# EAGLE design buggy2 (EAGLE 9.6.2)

## Sheet 1 of 2: MCU and power
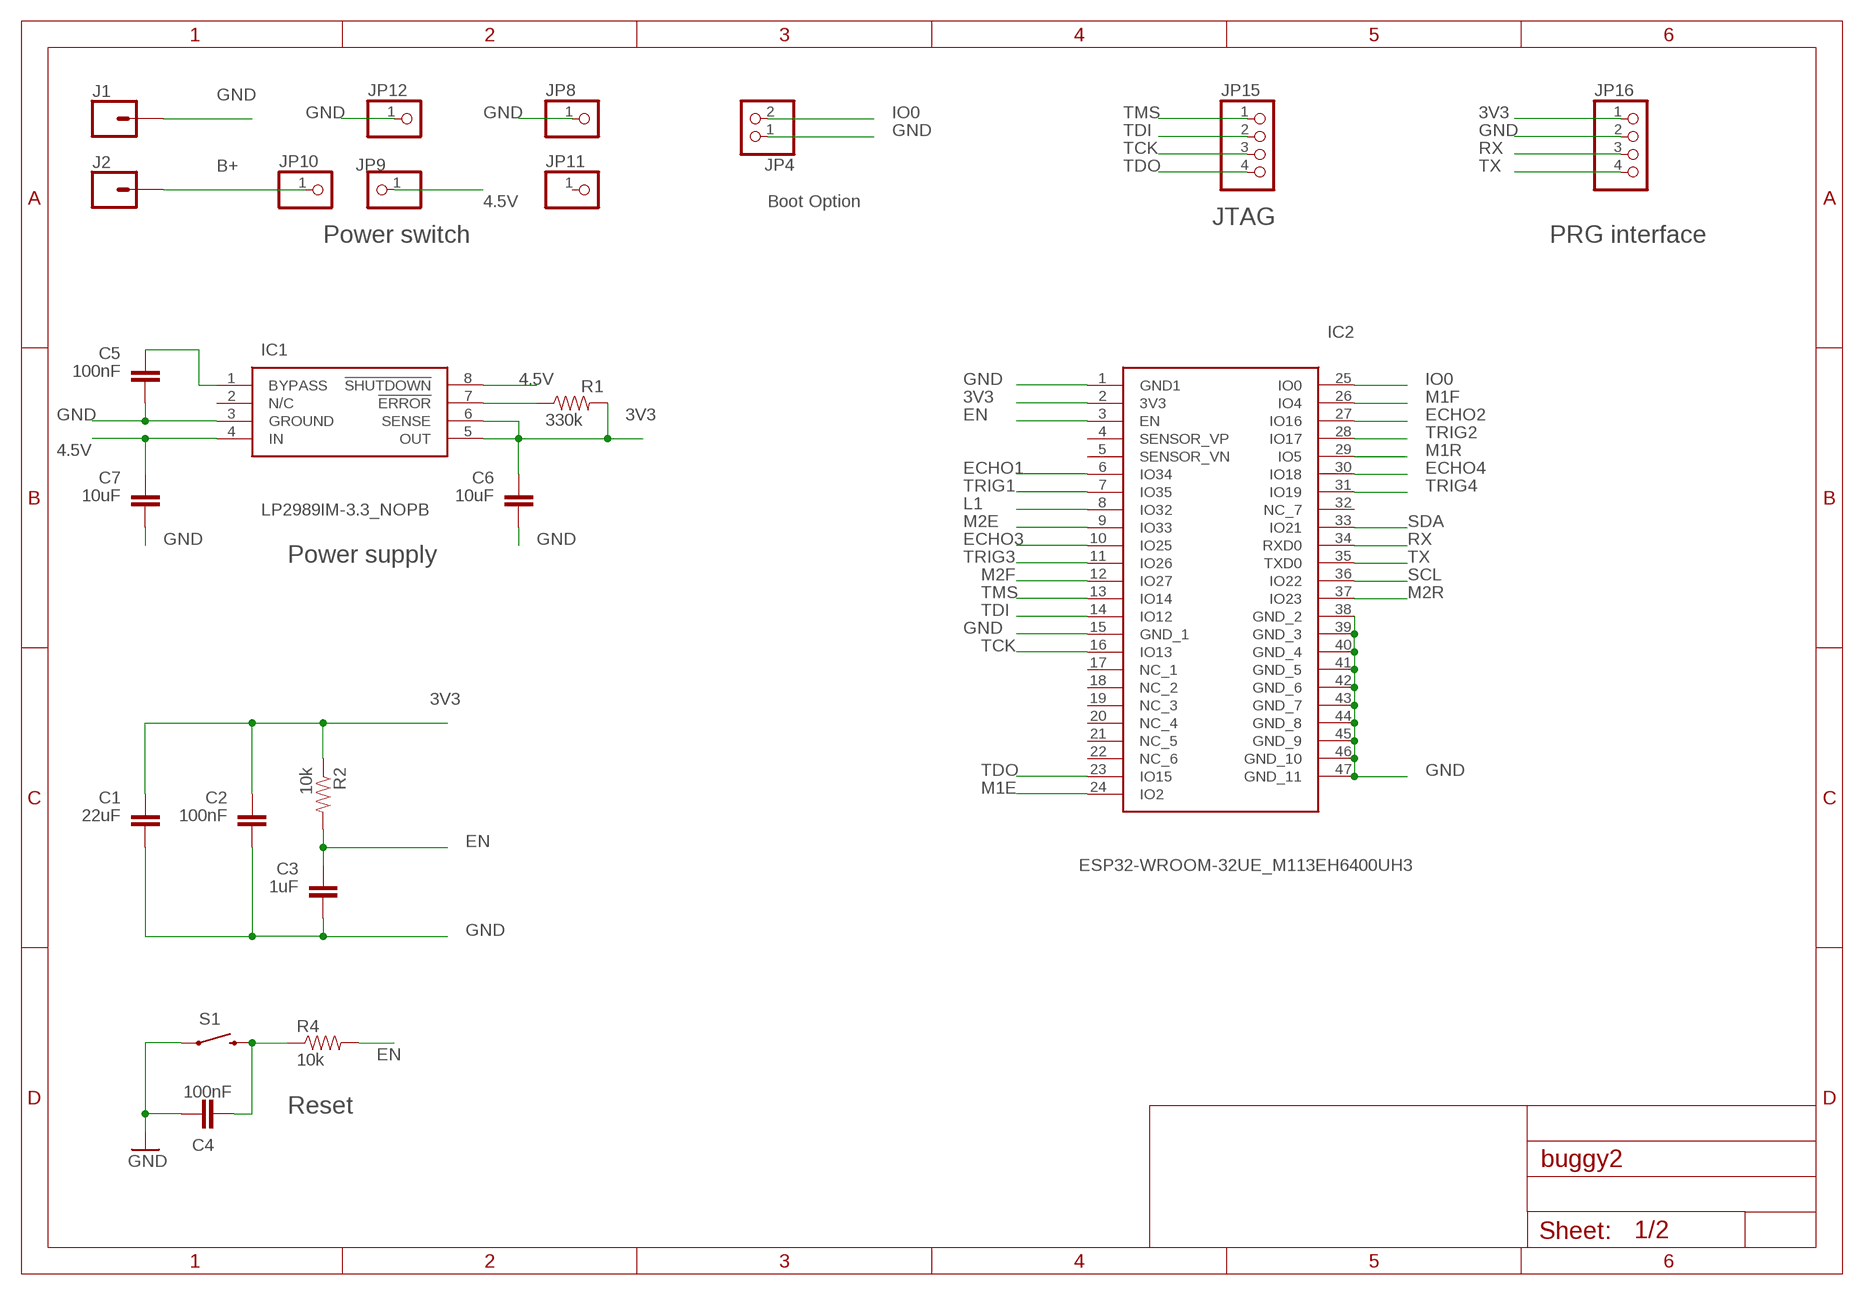
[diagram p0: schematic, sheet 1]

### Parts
C1  22uF  CAP0805  [0805]
C2  100nF  CAP0805  [0805]
C3  1uF  CAP0805  [0805]
C4  100nF  CAP0805  [0805]
C5  100nF  CAP0805  [0805]
C6  10uF  CAP0805  [0805]
C7  10uF  CAP0805  [0805]
IC1  LP2989IM-3.3_NOPB  [SOIC127P600X175-8N]
IC2  ESP32-WROOM-32UE_M113EH6400UH3  [ESP32WROOM32UEM113EH6400UH3Q0]
J1  CONN_01PTH_2MM  [1X01_2MM]
J2  CONN_01PTH_2MM  [1X01_2MM]
JP4  PINHD-1X2  [1X02]
JP8  PINHD-1X1  [1X01]
JP9  PINHD-1X1  [1X01]
JP10  PINHD-1X1  [1X01]
JP11  PINHD-1X1  [1X01]
JP12  PINHD-1X1  [1X01]
JP15  PINHD-1X4  [1X04]
JP16  PINHD-1X4  [1X04]
R1  330k  RESISTOR0805-RES  [0805]
R2  10k  RESISTOR0805-RES  [0805]
R4  10k  RESISTOR0805-RES  [0805]
S1  RESET  SWITCH-MOMENTARY-2SMD-1101NE  [TACTILE-SWITCH-1101NE]

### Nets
3V3: C1.1 C2.1 C6.1 IC1.5(OUT) IC1.6(SENSE) IC2.2(3V3) JP16.1 R1.2 R2.1 ; also sheet 2
4.5V: C7.1 IC1.4(IN) IC1.8(!SHUTDOWN) JP9.1 ; also sheet 2
B+: J2.1 JP10.1
ECHO1: IC2.6(IO34) ; also sheet 2
ECHO2: IC2.27(IO16) ; also sheet 2
ECHO3: IC2.10(IO25) ; also sheet 2
ECHO4: IC2.30(IO18) ; also sheet 2
EN: C3.1 IC2.3(EN) R2.2 R4.2
GND: C1.2 C2.2 C3.2 C4.1 C5.2 C6.2 C7.2 IC1.3(GROUND) IC2.1(GND1) IC2.15(GND_1) IC2.38(GND_2) IC2.39(GND_3) IC2.40(GND_4) IC2.41(GND_5) IC2.42(GND_6) IC2.43(GND_7) IC2.44(GND_8) IC2.45(GND_9) IC2.46(GND_10) IC2.47(GND_11) J1.1 JP4.1 JP8.1 JP12.1 JP16.2 S1.1 ; also sheet 2
IO0: IC2.25(IO0) JP4.2
L1: IC2.8(IO32) ; also sheet 2
M1E: IC2.24(IO2) ; also sheet 2
M1F: IC2.26(IO4) ; also sheet 2
M1R: IC2.29(IO5) ; also sheet 2
M2E: IC2.9(IO33) ; also sheet 2
M2F: IC2.12(IO27) ; also sheet 2
M2R: IC2.37(IO23) ; also sheet 2
N$1: C5.1 IC1.1(BYPASS)
N$3: C4.2 R4.1 S1.2
N$18: IC1.7(!ERROR) R1.1
RX: IC2.34(RXD0) JP16.3
SCL: IC2.36(IO22) ; also sheet 2
SDA: IC2.33(IO21) ; also sheet 2
TCK: IC2.16(IO13) JP15.3
TDI: IC2.14(IO12) JP15.2
TDO: IC2.23(IO15) JP15.4
TMS: IC2.13(IO14) JP15.1
TRIG1: IC2.7(IO35) ; also sheet 2
TRIG2: IC2.28(IO17) ; also sheet 2
TRIG3: IC2.11(IO26) ; also sheet 2
TRIG4: IC2.31(IO19) ; also sheet 2
TX: IC2.35(TXD0) JP16.4
Unconnected: IC1.2(N/C) IC2.4(SENSOR_VP) IC2.5(SENSOR_VN) IC2.17(NC_1) IC2.18(NC_2) IC2.19(NC_3) IC2.20(NC_4) IC2.21(NC_5) IC2.22(NC_6) IC2.32(NC_7) JP11.1

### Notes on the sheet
- Boot Option
- JTAG
- Power switch | PRG interface
- Power supply
- Reset

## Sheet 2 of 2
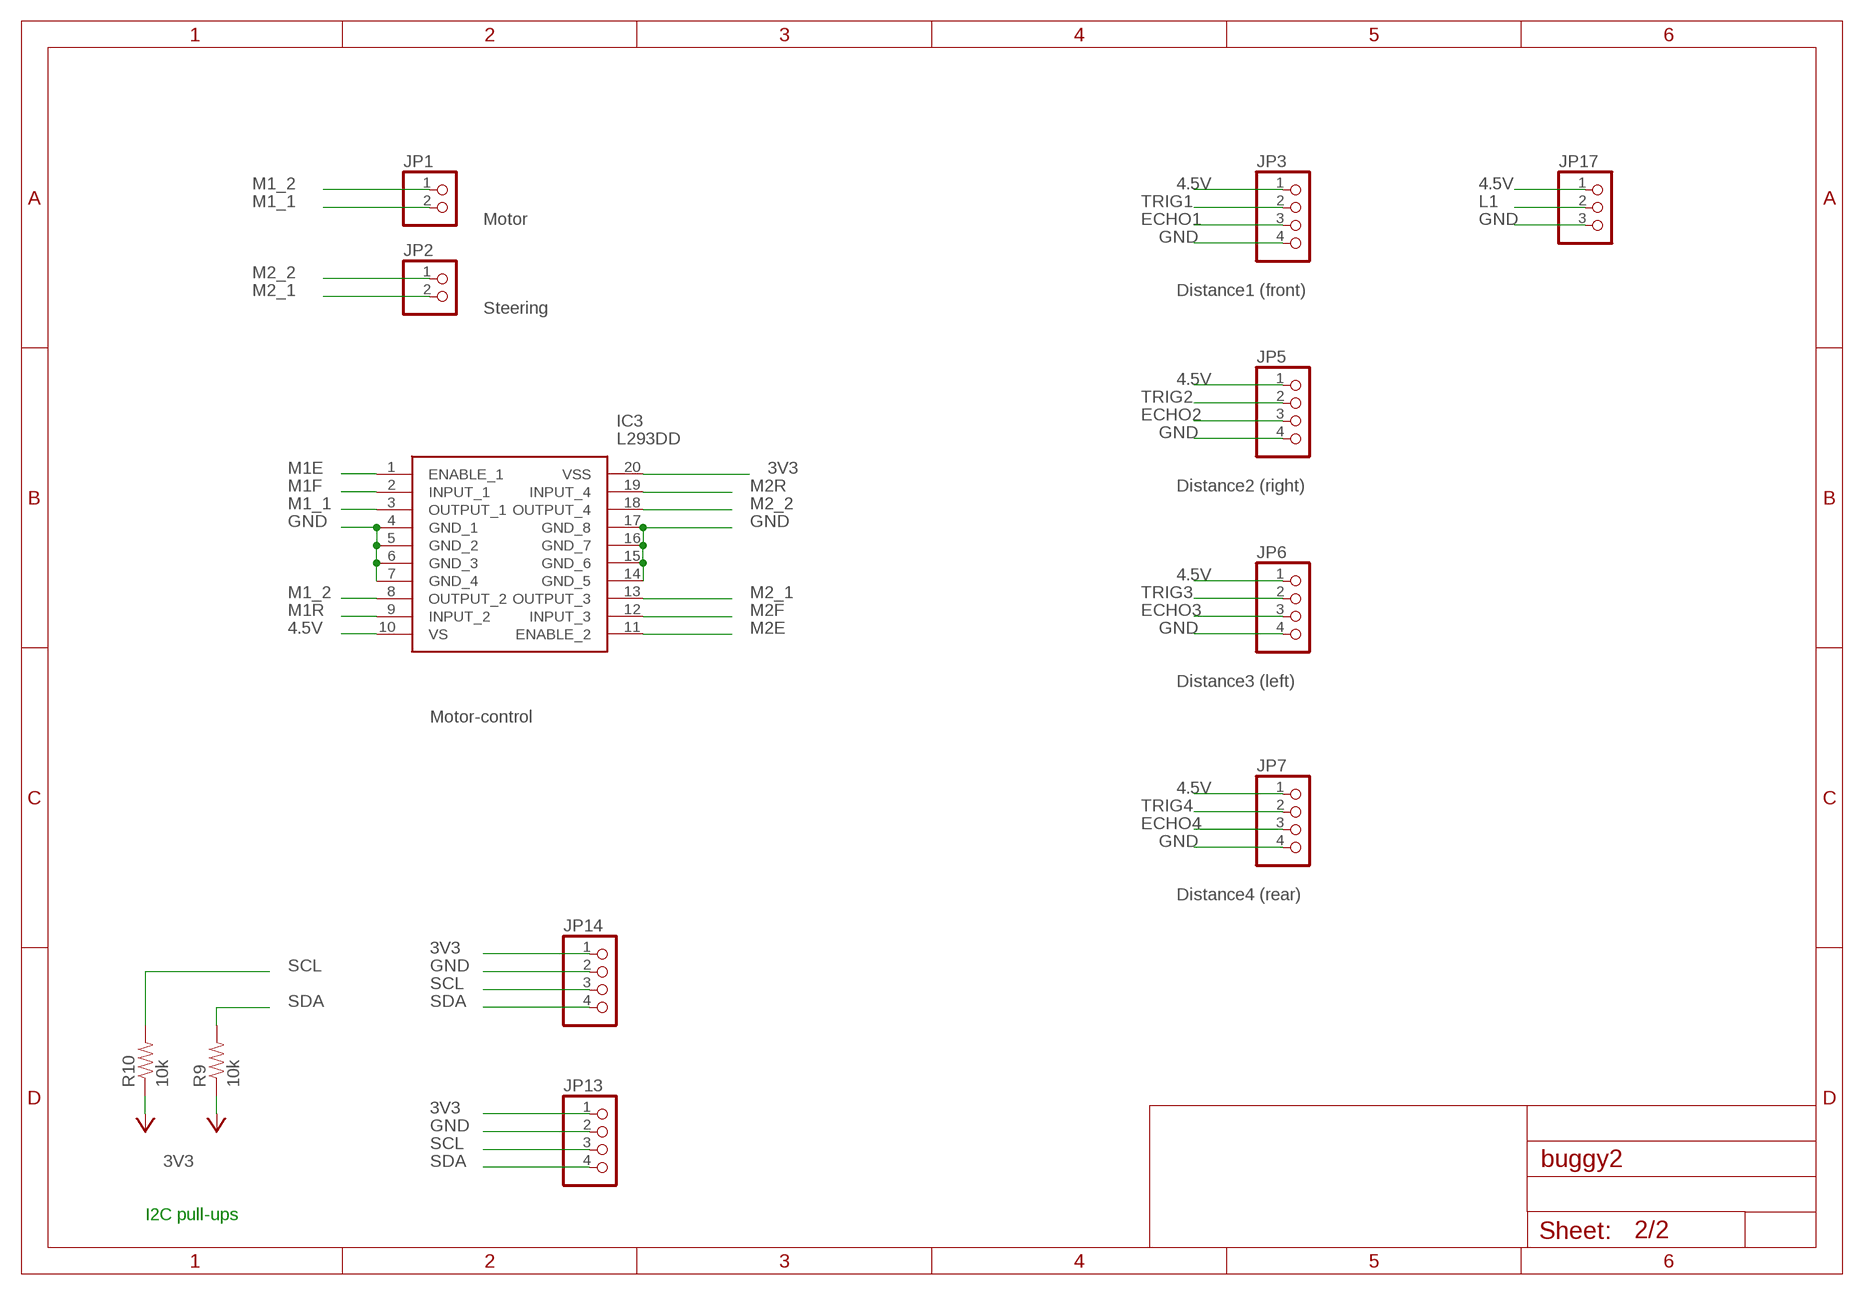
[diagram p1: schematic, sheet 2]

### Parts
IC3  L293DD  [SOIC127P1032X265-20N]
JP1  PINHD-1X2/90  [1X02/90]
JP2  PINHD-1X2/90  [1X02/90]
JP3  PINHD-1X4  [1X04]
JP5  PINHD-1X4  [1X04]
JP6  PINHD-1X4  [1X04]
JP7  PINHD-1X4  [1X04]
JP13  PINHD-1X4  [1X04]
JP14  PINHD-1X4  [1X04]
JP17  PINHD-1X3  [1X03]
R9  10k  RESISTOR0805-RES  [0805]
R10  10k  RESISTOR0805-RES  [0805]

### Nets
3V3: IC3.20(VSS) JP13.1 JP14.1 R9.1 R10.1 ; supply symbol labelled +3V3 ; also sheet 1
4.5V: IC3.10(VS) JP3.1 JP5.1 JP6.1 JP7.1 JP17.1 ; also sheet 1
ECHO1: JP3.3 ; also sheet 1
ECHO2: JP5.3 ; also sheet 1
ECHO3: JP6.3 ; also sheet 1
ECHO4: JP7.3 ; also sheet 1
GND: IC3.4(GND_1) IC3.5(GND_2) IC3.6(GND_3) IC3.7(GND_4) IC3.14(GND_5) IC3.15(GND_6) IC3.16(GND_7) IC3.17(GND_8) JP3.4 JP5.4 JP6.4 JP7.4 JP13.2 JP14.2 JP17.3 ; also sheet 1
L1: JP17.2 ; also sheet 1
M1_1: IC3.3(OUTPUT_1) JP1.2
M1_2: IC3.8(OUTPUT_2) JP1.1
M1E: IC3.1(ENABLE_1) ; also sheet 1
M1F: IC3.2(INPUT_1) ; also sheet 1
M1R: IC3.9(INPUT_2) ; also sheet 1
M2_1: IC3.13(OUTPUT_3) JP2.2
M2_2: IC3.18(OUTPUT_4) JP2.1
M2E: IC3.11(ENABLE_2) ; also sheet 1
M2F: IC3.12(INPUT_3) ; also sheet 1
M2R: IC3.19(INPUT_4) ; also sheet 1
SCL: JP13.3 JP14.3 R10.2 ; also sheet 1
SDA: JP13.4 JP14.4 R9.2 ; also sheet 1
TRIG1: JP3.2 ; also sheet 1
TRIG2: JP5.2 ; also sheet 1
TRIG3: JP6.2 ; also sheet 1
TRIG4: JP7.2 ; also sheet 1

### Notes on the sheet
- Motor
- Distance1 (front)
- Steering
- Distance2 (right)
- Distance3 (left)
- Motor-control
- Distance4 (rear)
- I2C pull-ups

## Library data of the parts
C1-C7 = SparkFun-Passives:CAP: Capacitor
IC1 = SamacSys_Parts:LP2989IM-3.3_NOPB: Micropower/Low Noise, 500 mA Ultra Low-Dropout Regulator Source: Datasheet; DESCRIPTION: Micropower/Low Noise, 500 mA Ultra Low-Dropout Regulator; HEIGHT: 1.75mm; MANUFACTURER_NAME: Texas Instruments; MANUFACTURER_PART_NUMBER: LP2989IM-3.3/NOPB; MOUSER_PART_NUMBER: 926-2989IM-3.3/NOPB; MOUSER_PRICE-STOCK: https://www.mouser.co.uk/ProductDetail/Texas-Instruments/LP2989IM-33-NOPB?qs=1FNqv8aZn1Tm79MYQqSiDQ%3D%3D
IC2 = SamacSys_Parts:ESP32-WROOM-32UE_M113EH6400UH3: WiFi Modules (802.11) SMD module ESP32-WROOM-32UE, ESP32-D0WD-V3, ESP32 ECO V3, 8 MB SPI flash, IPEX antenna connector Source: Datasheet; DESCRIPTION: WiFi Modules (802.11) SMD module ESP32-WROOM-32UE, ESP32-D0WD-V3, ESP32 ECO V3, 8 MB SPI flash, IPEX antenna connector; HEIGHT: 3.35mm; MANUFACTURER_NAME: Espressif Systems; MANUFACTURER_PART_NUMBER: ESP32-WROOM-32UE(M113EH6400UH3Q0); MOUSER_PART_NUMBER: 356-ESP32WRM32UE64UH; MOUSER_PRICE-STOCK: https://www.mouser.co.uk/ProductDetail/Espressif-Systems/ESP32-WROOM-32UEM113EH6400UH3Q0?qs=vHuUswq2%252BsxjtHWnhz9C5Q%3D%3D
IC3 = SamacSys_Parts:L293DD: L293DD, Motor Driver, 4.5 36 V, 20-Pin SOIC Source: Datasheet; DESCRIPTION: L293DD, Motor Driver, 4.5 36 V, 20-Pin SOIC; HEIGHT: 2.65mm; MANUFACTURER_NAME: STMicroelectronics; MANUFACTURER_PART_NUMBER: L293DD; MOUSER_PART_NUMBER: 511-L293DD; MOUSER_PRICE-STOCK: https://www.mouser.co.uk/ProductDetail/STMicroelectronics/L293DD?qs=m4gxtLzGBzoksItTiSkcgg%3D%3D
J1 J2 = SparkFun-Connectors:CONN_01: Single connection point. Often used as Generic Header-pin footprint for 0.1 inch spaced/style header connections
JP1 JP2 JP4 = pinhead:PINHD-1X2: PIN HEADER
JP3 JP5-JP7 JP13-JP16 = pinhead:PINHD-1X4: PIN HEADER
JP8-JP12 = pinhead:PINHD-1X1: PIN HEADER
JP17 = pinhead:PINHD-1X3: PIN HEADER
R1 R2 R4 R9 R10 = SparkFun-Resistors:RESISTOR: Resistor
S1 = SparkFun-Electromechanical:SWITCH-MOMENTARY-2: Various NO switches- pushbuttons, reed, etc; PROD_ID: SWCH-00815

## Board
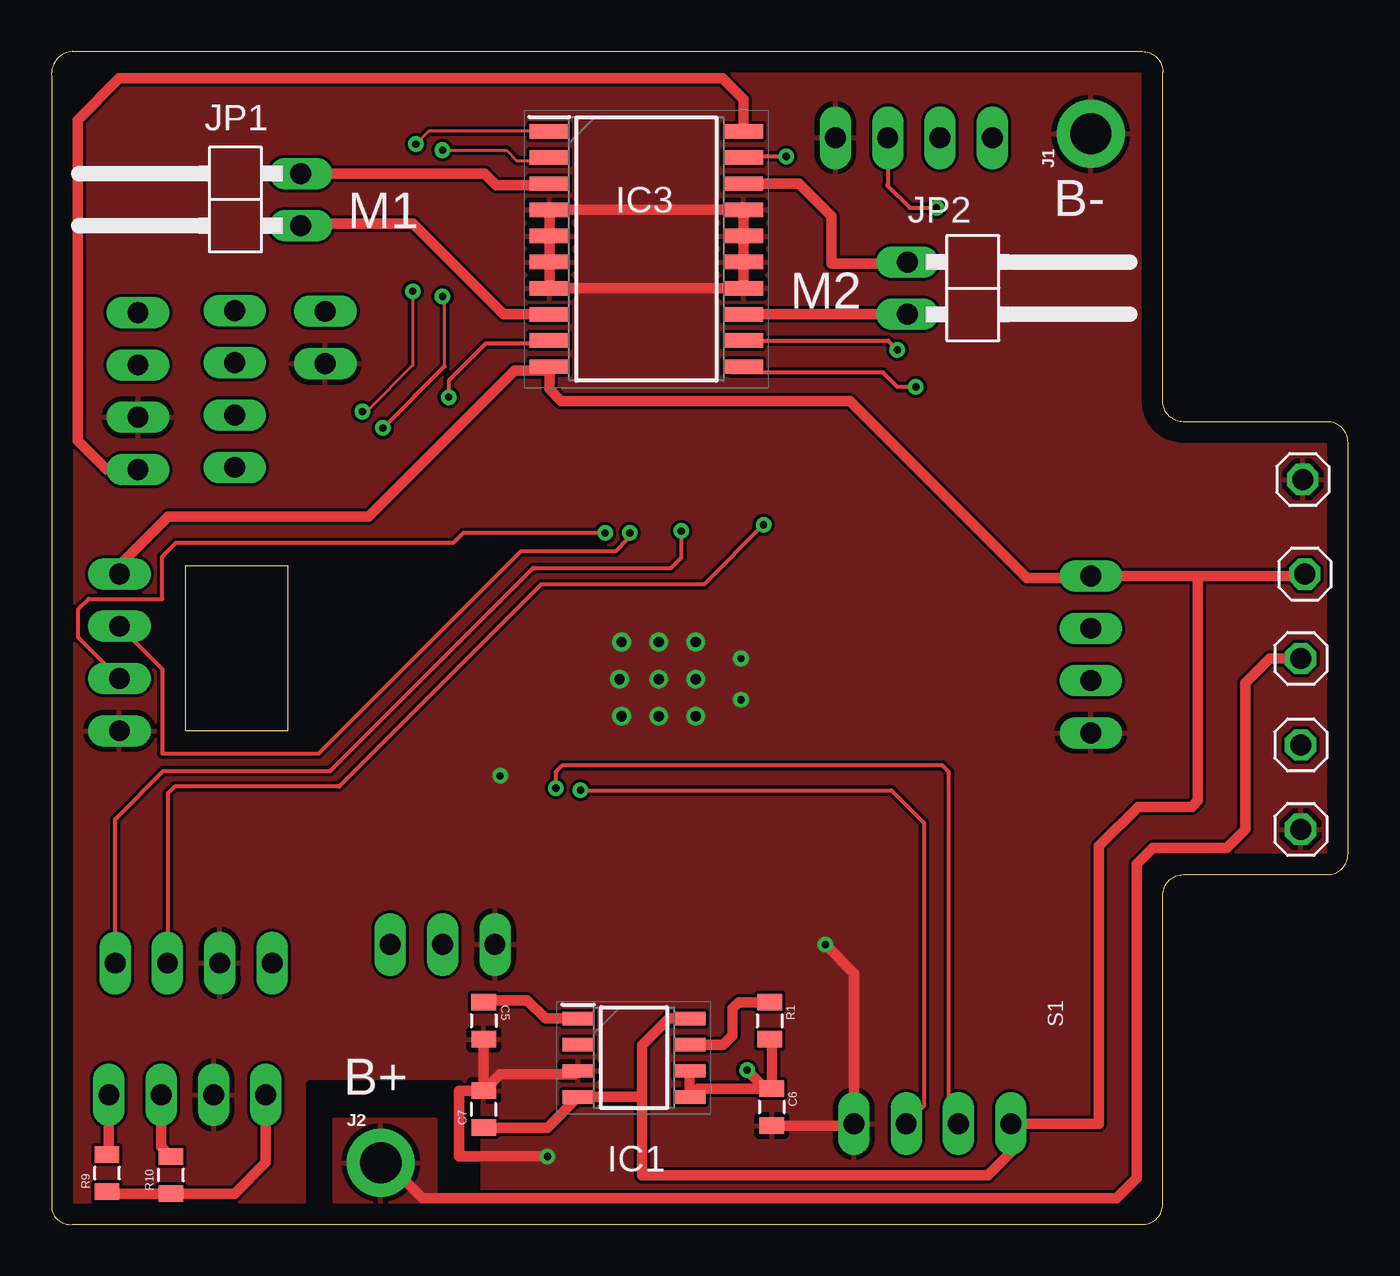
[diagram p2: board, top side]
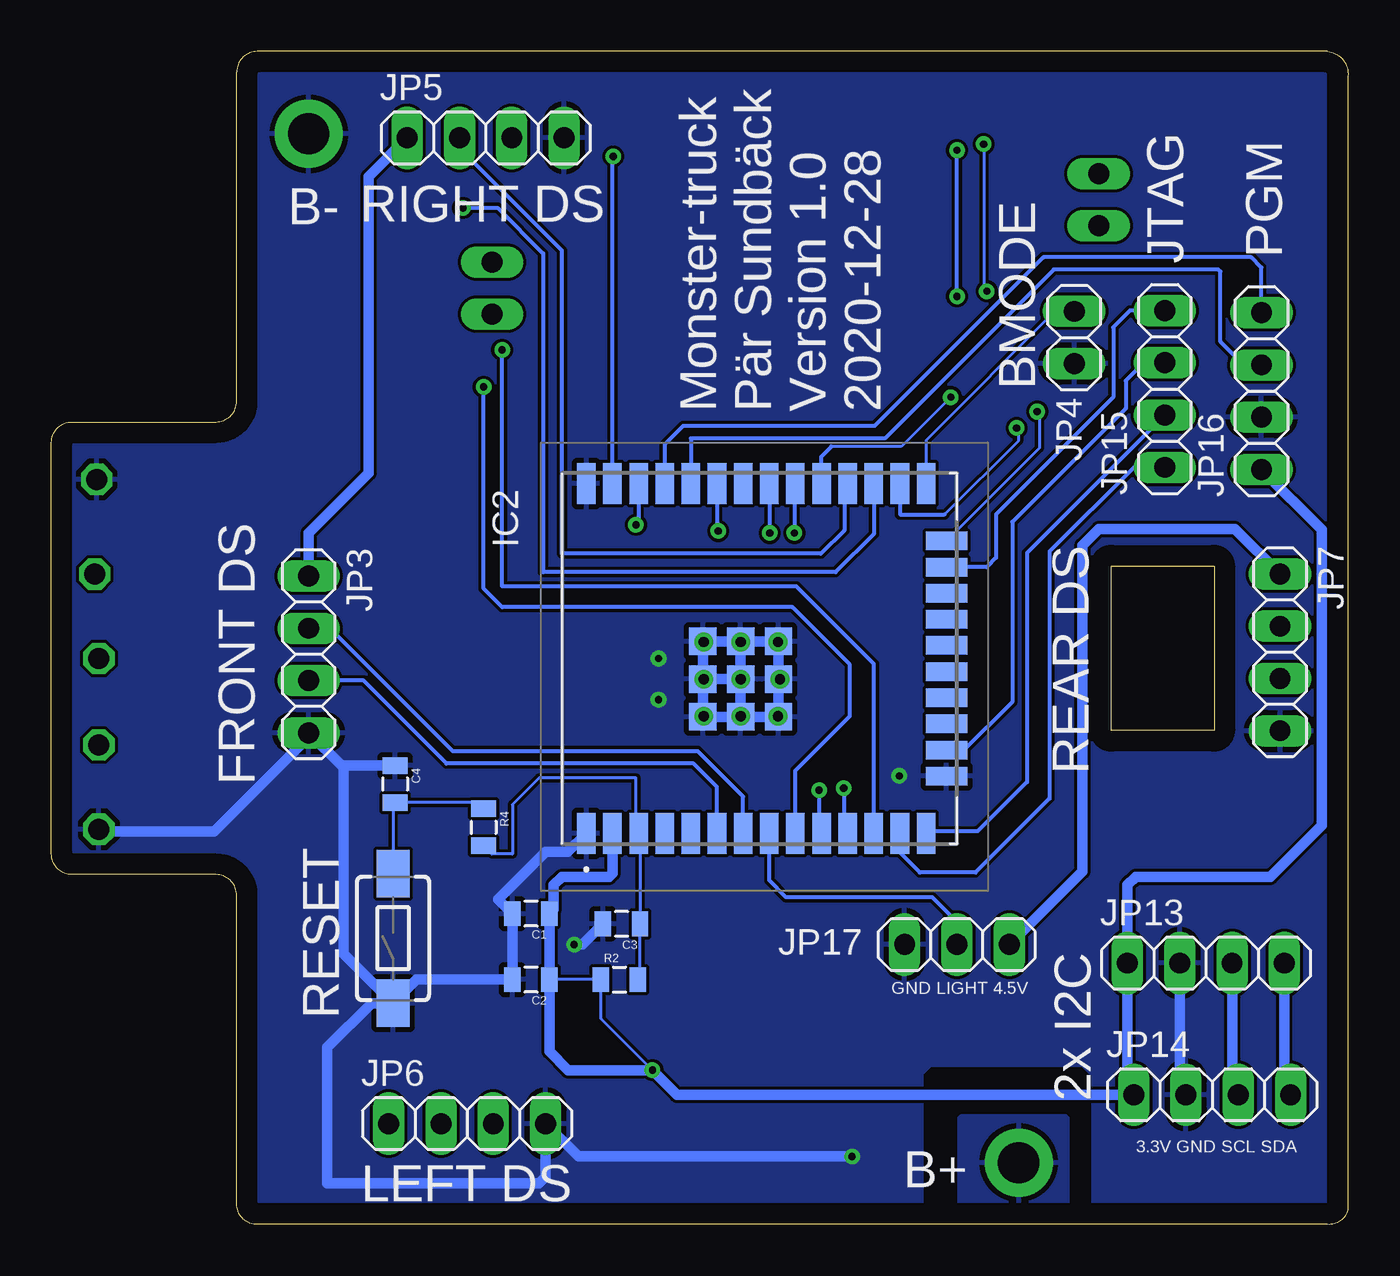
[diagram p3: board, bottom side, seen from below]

Size 63 x 57.01 mm. Coordinates in mm from the lower left corner, seen from the top.
Outline: 0,55.81 0,0.81 arc90 1,0.01 53,0.01 arc90 54,1.01 54,16.01 arc-90 55,17.01 62,17.01 arc90 63,18.01 63,38.01 arc90 62,39.01 55,39.01 arc-90 54,40.01 54,56.01 arc90 53,57.01 1,57.01 arc90 0,55.81
Outline: 6.5,32.01 6.5,24.01 11.5,24.01 11.5,32.01 6.5,32.01
Copper layers (1*16): Top 0.035mm / dielectric 1.5mm / Bottom 0.035mm
Design rules "default": minimum track width 6mil, minimum drill 0.35mm, track to track 6mil, track to pad 6mil, pad to pad 6mil, via to via 6mil, smd to smd 6mil, copper to edge 40mil, drill to drill 6mil, minimum pad ring 10mil, minimum via ring 8mil, stop-mask expansion 4mil, vias tented up to drill 0mil, thermal gap 10mil

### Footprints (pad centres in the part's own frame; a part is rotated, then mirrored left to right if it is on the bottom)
0805 = smd 0.8 x 1.2: 1 -0.9,0; 2 0.9,0
SOIC127P600X175-8N = smd 1.528 x 0.65: 1 -2.711,1.905; 2 -2.711,0.635; 3 -2.711,-0.635; 4 -2.711,-1.905; 5 2.711,-1.905; 6 2.711,-0.635; 7 2.711,0.635; 8 2.711,1.905
ESP32WROOM32UEM113EH6400UH3Q0 = smd 2 x 0.9: 1 -8.5,8.41; 2 -8.5,7.14; 3 -8.5,5.87; 4 -8.5,4.6; 5 -8.5,3.33; 6 -8.5,2.06; 7 -8.5,0.79; 8 -8.5,-0.48; 9 -8.5,-1.75; 10 -8.5,-3.02; 11 -8.5,-4.29; 12 -8.5,-5.56; 13 -8.5,-6.83; 14 -8.5,-8.1; 25 8.5,-8.1; 26 8.5,-6.83; 27 8.5,-5.56; 28 8.5,-4.29; 29 8.5,-3.02; 30 8.5,-1.75; 31 8.5,-0.48; 32 8.5,0.79; 33 8.5,2.06; 34 8.5,3.33; 35 8.5,4.6; 36 8.5,5.87; 37 8.5,7.14; 38 8.5,8.41 | smd 0.9 x 2: 15 -5.715,-9.1; 16 -4.445,-9.1; 17 -3.175,-9.1; 18 -1.905,-9.1; 19 -0.635,-9.1; 20 0.635,-9.1; 21 1.905,-9.1; 22 3.175,-9.1; 23 4.445,-9.1; 24 5.715,-9.1 | smd 1.33 x 1.33: 39 -1,0.91; 40 0.835,0.91; 41 0.835,2.745; 42 -1,2.745; 43 -2.835,2.745; 44 -2.835,0.91; 45 -2.835,-0.925; 46 -1,-0.925; 47 0.835,-0.925
SOIC127P1032X265-20N = smd 1.925 x 0.7: 1 -4.712,5.715; 2 -4.712,4.445; 3 -4.712,3.175; 4 -4.712,1.905; 5 -4.712,0.635; 6 -4.712,-0.635; 7 -4.712,-1.905; 8 -4.712,-3.175; 9 -4.712,-4.445; 10 -4.712,-5.715; 11 4.712,-5.715; 12 4.712,-4.445; 13 4.712,-3.175; 14 4.712,-1.905; 15 4.712,-0.635; 16 4.712,0.635; 17 4.712,1.905; 18 4.712,3.175; 19 4.712,4.445; 20 4.712,5.715
1X01_2MM = drill 2 pad 3.302: 1 0,0
1X02/90 = drill 1.016 long: 1 -1.27,-3.81; 2 1.27,-3.81
1X04 = drill 1.016 long: 1 -3.81,0; 2 -1.27,0; 3 1.27,0; 4 3.81,0
1X02 = drill 1.016 long: 1 -1.27,0; 2 1.27,0
1X01 = drill 1.016 octagon: 1 0,0
1X03 = drill 1.016 long: 1 -2.54,0; 2 0,0; 3 2.54,0
TACTILE-SWITCH-1101NE = smd 2.3 x 1.6: 1 -3.15,0; 2 3.15,0

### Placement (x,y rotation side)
C1  39.7,15.11 180 bottom
C2  39.7,11.91 180 bottom
C3  35.3,14.61 180 bottom
C4  46.3,21.41 270 bottom
C5  21,9.91 270.3 top
C6  35,5.71 270 top
C7  21,5.61 90 top
IC1  28.3,8.11 0 top
IC2  28.6,27.51 90 bottom
IC3  28.9,47.41 0 top
J1  50.5,53.01 90 top
J2  16,3.01 0 top
JP1  8.3,49.81 90 top
JP2  45.4,45.51 270 top
JP3  50.5,27.71 270 bottom
JP4  13.3,43.11 90 bottom
JP5  41.9,52.81 0 bottom
JP6  42.8,4.91 0 bottom
JP7  3.3,27.81 270 bottom
JP8  60.8,36.21 0 top
JP9  60.9,31.61 0 top
JP10  60.7,27.51 0 top
JP11  60.7,23.31 0 top
JP12  60.7,19.21 0 top
JP13  6.9,12.71 0 bottom
JP14  6.6,6.31 0 bottom
JP15  8.9,40.61 90 bottom
JP16  4.2,40.51 90 bottom
JP17  19,13.61 180 bottom
R1  34.9,9.91 270 top
R2  35.4,11.91 0 bottom
R4  42,19.31 270 bottom
R9  2.7,2.51 90 top
R10  5.8,2.41 90 top
S1  46.4,13.91 90 bottom

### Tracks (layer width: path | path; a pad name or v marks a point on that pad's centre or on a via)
3V3  (via drill 0.35)
  Top 0.508: IC1.6 IC1.5 31.42,6.61 C6.1 | R1.2 35,8.91 C6.1 | v33.8,7.51 34.7,6.61 C6.1 | R9.1 2.8,1.51 R10.1 8.9,1.51 10.41,3.02 JP14.1 | JP16.1 2.68,36.7 1.27,38.11 1.27,53.68 3.3,55.71 32.6,55.71 33.62,54.69 IC3.20
  Bottom 0.152: 38.8,12.01 C2.1 R2.1 36.3,10.01 v33.8,7.51
  Bottom 0.508: 38.8,12.01 38.8,8.41 37.9,7.51 v33.8,7.51 32.6,6.31 JP14.1 10.71,6.61 JP13.1 10.71,16.5 10.3,16.91 3.77,16.91 1.27,19.41 1.27,33.77 JP16.1 | C2.1 C1.1 38.6,15.31 38.6,16.51 38.2,16.91 35.9,16.91 35.74,17.07 IC2.2
4.5V
  Top 0.508: 28.7,6.21 28.7,2.41 45.51,2.41 46.61,3.51 JP6.1 50.9,4.91 50.9,18.41 52.8,20.31 55.4,20.31 55.7,20.61 55.7,31.52 | 28.7,6.21 28.7,8.71 30.01,10.01 IC1.8 | 28.7,6.21 IC1.4 24.1,4.71 C7.1 | IC3.10 24.19,41.51 | 24.19,41.51 24.19,40.59 24.77,40.01 38.8,40.01 47.4,31.41 50.39,31.41 JP3.1 55.7,31.52 | JP7.1 3.23,31.69 3.23,31.98 5.66,34.41 15.4,34.41 22.5,41.51 24.19,41.51 | 55.7,31.52 60.81,31.52 JP9.1
  Bottom 0.508: JP5.1 47.6,50.92 47.6,36.51 50.5,33.61 JP3.1 | JP17.1 12.9,17.17 12.9,33.01 12.1,33.81 5.49,33.81 JP7.1
B+
  Top 0.508: J2.1 16.3,3.01 18.03,1.28 51.73,1.28 52.73,2.28 52.73,17.53 53.51,18.31 57.1,18.31 58,19.21 58,26.31 59.2,27.51 JP10.1
  pour Top: 13.7,5.11 13.7,1.11 18.7,1.11 18.7,5.11
  pour Bottom: 13.6,5.21 13.6,0.91 18.8,0.91 18.9,1.01 18.9,5.21 18.8,5.31 13.7,5.31
ECHO1
  Bottom 0.2: IC2.6 30.66,21.27 31.8,22.41 43.8,22.41 47.83,26.44 JP3.3
ECHO2  (via drill 0.35)
  Top 0.2: JP5.3 40.63,50.54 40.6,50.51 41.7,49.41 v43,49.41
  Bottom 0.2: IC2.27 23.04,33.57 24.9,31.71 39.1,31.71 39.1,47.18 41.33,49.41 v43,49.41
ECHO3  (via drill 0.35)
  Top 0.2: v25.7,21.11 40.8,21.11 42.4,19.51 42.4,5.78 JP6.3
  Bottom 0.2: v25.7,21.11 25.7,19.13 IC2.10
ECHO4  (via drill 0.35)
  Top 0.2: JP7.3 1.3,28.54 1.3,29.91 1.8,30.41 5.39,30.41 5.39,32.47 6.04,33.12 19.52,33.12 20,33.61 v26.9,33.61
  Bottom 0.2: IC2.30 26.9,35.96 v26.9,33.61
EN
  Bottom 0.152: R2.2 34.4,12.01 C3.1 34.4,19.01 IC2.3 34.6,19.14 34.6,21.71 39.3,21.71 40.6,20.41 40.6,18.01 41.6,18.01 R4.2
GND  (via drill 0.35, 0.5)
  Top 0.508: C5.2 C7.2 | C7.2 19.8,6.51 19.8,3.31 v24.1,3.31 | IC1.3 25.43,7.31 21.8,7.31 C7.2 | C6.2 38.89,4.81 JP6.4 38.99,12.22 v37.6,13.61 | IC3.4 IC3.5 IC3.6 IC3.7 IC3.14 IC3.15 IC3.16 IC3.17 IC3.4
  Bottom 0.508: JP13.2 8.17,6.61 JP14.2 | S1.1 47.45,10.76 49.6,8.61 49.6,2.01 39.3,2.01 38.99,2.32 JP6.4 37.39,3.31 v24.1,3.31 | S1.1 45.25,11.91 C2.2 C1.2 41.3,15.81 39,18.11 37.91,18.11 IC2.1 | 48.8,22.31 48.91,22.31 JP3.4 50.5,23.71 55.1,19.11 60.6,19.11 JP12.1 | 48.8,22.31 C4.1 | v37.6,13.61 37.2,13.61 C3.2 | S1.1 48.8,13.16 48.8,22.31 | IC2.40 IC2.47 IC2.46 IC2.45 IC2.44 | IC2.40 IC2.41 IC2.42 | IC2.42 IC2.43 IC2.44 | IC2.39 IC2.44 | IC2.40 IC2.39 | IC2.39 IC2.42
  other vias: 21.8,21.81 31.3,28.31 27.6,26.51 27.7,28.31 29.5,28.31 29.5,26.51 31.3,26.51 27.7,24.71 29.5,24.71 31.3,24.71 33.5,27.51 33.5,25.51
  pour Top: -1.1,56.31 -1.1,0.81 0.7,-0.99 10.6,-0.99 10.9,-0.69 12.3,0.71 12.3,6.91 12.5,7.11 19.9,7.11 20.9,6.11 20.9,-0.59 21.4,-1.09 54.3,-1.09 64.6,9.21 64.6,54.11 60.7,58.01 0.1,58.01 -1.1,56.81
  pour Bottom: -2,57.31 -2,-1.19 -2.1,-1.29 12.1,-1.29 12.4,-0.99 12.4,7.21 12.9,7.71 20.3,7.71 20.7,7.31 20.7,-1.29 56.1,-1.29 56.4,-0.99 64.6,7.21 64.6,24.11 64.6,57.01 62.9,58.71 -0.6,58.71
IO0
  Bottom 0.152: JP4.2 14.23,44.38 20.5,38.11 IC2.25
L1
  Bottom 0.2: JP17.2 19,14.71 20.2,15.91 27.3,15.91 28.12,16.73 IC2.8
M1_1
  Top 0.508: JP1.2 21.03,51.08 21.6,50.51 24.12,50.51 IC3.3
M1_2
  Top 0.508: IC3.8 21.98,44.23 17.57,48.64 12.21,48.64 JP1.1
M1E  (via drill 0.35)
  Top 0.152: IC3.1 18.32,53.12 v17.7,52.51 | v17.55,45.36 17.55,41.76 15.3,39.51 v15.1,39.51
  Bottom 0.152: v17.7,52.51 17.7,45.41 17.6,45.31 v17.55,45.36 | v15.1,39.51 15,39.41 15,37.72 IC2.24
M1F  (via drill 0.35)
  Top 0.152: 19.1,41.71 19.1,45.11 v19,45.11 | v19,52.21 22.1,52.21 22.6,51.71 24.05,51.71 IC3.2
  Top 0.2: v16.1,38.71 19.1,41.71
  Bottom 0.152: v16.1,38.71 16,38.61 16,38.11 19.6,34.51
  Bottom 0.2: IC2.26 21.77,34.51 19.6,34.51 | v19,45.11 v19,52.21
M1R  (via drill 0.35)
  Top 0.152: IC3.9 24.04,42.81
  Top 0.2: 24.04,42.81 21.1,42.81 19.3,41.01 v19.3,40.21
  Bottom 0.152: v19.3,40.21 21.7,37.81 25.1,37.81 | 25.6,36.03 IC2.29
  Bottom 0.2: 25.1,37.81 25.6,37.31 25.6,36.03
M2_1
  Top 0.508: IC3.13 37.59,44.23 37.59,44.24 JP2.2
M2_2
  Top 0.508: IC3.18 36.33,50.58 37.9,49.01 37.9,46.71 41.52,46.71 JP2.1
M2E  (via drill 0.35)
  Top 0.2: v42,40.71 41.1,40.71 40.4,41.41 33.03,41.41 33.32,41.69 IC3.11
  Bottom 0.2: IC2.9 26.85,22.06 24.2,24.71 24.2,27.21 27,30.01 41.1,30.01 42,30.91 v42,40.71
M2F  (via drill 0.35)
  Top 0.2: IC3.12 40.65,42.96 v41.1,42.51
  Bottom 0.2: IC2.12 23.04,27.25 26.8,31.01 41.1,31.01 v41.1,42.51
M2R  (via drill 0.35)
  Top 0.2: IC3.19 33.67,51.91 v35.7,51.91
  Bottom 0.2: IC2.37 35.74,51.87 v35.7,51.91
N$1
  Top 0.508: IC1.1 24,10.01 23.1,10.91 21.1,10.91 C5.1
N$3
  Bottom 0.152: S1.2 46.4,20.41 C4.2 42.3,20.51 R4.1
N$18
  Top 0.508: IC1.7 32.64,8.74 33.1,9.21 33.1,10.51 33.4,10.81 R1.1
RX
  Bottom 0.2: JP16.3 5.07,41.78 6.2,42.91 6.2,46.31 6.3,46.41 14.3,46.41 22.5,38.21 31.93,38.21 IC2.34
SCL  (via drill 0.35)
  Top 0.2: v34.6,34.01 31.7,31.11 23.8,31.11 13.98,21.28 5.98,21.28 5.65,20.96 5.65,12.73 JP13.3
  Top 0.508: JP14.3 5.33,3.78 R10.2
  Bottom 0.2: IC2.36 34.47,34.14 v34.6,34.01
  Bottom 0.508: JP13.3 5.63,6.61 JP14.3
SDA  (via drill 0.35)
  Top 0.2: JP13.4 3.09,19.7 5.44,22.04 13.53,22.04 23.4,31.91 30.1,31.91 30.6,32.41 v30.6,33.71
  Top 0.508: JP14.4 2.79,3.5 R9.2
  Bottom 0.2: IC2.33 30.66,33.77 v30.6,33.71
  Bottom 0.508: JP13.4 3.09,6.61 JP14.4
TCK
  Bottom 0.2: JP15.3 9.93,41.88 10.8,41.01 10.8,39.66 16.32,34.14 16.32,25.39 18.7,23.01 19.45,23.01 IC2.16
TDI
  Bottom 0.2: JP15.2 15.6,32.64 15.6,21.51 18,19.11 20.4,19.11 IC2.14
TDO
  Bottom 0.2: JP15.4 10.59,44.42 11.4,43.61 11.4,40.21 17.1,34.51 17.1,32.41 17.56,31.95 IC2.23
TMS
  Bottom 0.2: JP15.1 10.4,36.8 14.5,32.7 14.5,20.71 18.1,17.11 20.8,17.11 21.77,18.08 IC2.13
TRIG1
  Bottom 0.2: JP3.2 50.43,28.91 49.4,28.91 43.5,23.01 31.6,23.01 29.39,20.8 IC2.7
TRIG2
  Bottom 0.2: IC2.28 24.48,35.84 24.48,33.74 25.61,32.61 38.2,32.61 38.2,47.34 43.17,52.31 JP5.2
TRIG3  (via drill 0.35)
  Top 0.2: JP6.2 43.6,5.38 43.6,22.01 43.3,22.31 24.8,22.31 24.5,22.01 v24.5,21.21
  Bottom 0.2: v24.5,21.21 24.5,19.2 IC2.11
TRIG4  (via drill 0.35)
  Top 0.2: JP7.2 5.39,26.99 5.39,22.89 12.99,22.89 22.8,32.71 27.4,32.71 28,33.31 28,33.51 v28.1,33.61
  Bottom 0.2: IC2.31 28.1,35.99 v28.1,33.61
TX
  Bottom 0.2: JP16.4 4.2,46.51 4.7,47.01 14.8,47.01 23,38.81 32.3,38.81 33.2,37.91 IC2.35

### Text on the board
tNames: B- | M1 | M2 | B+
bNames: RIGHT DS | B- | PGM | JTAG | BMODE | Monster-truck / Pär Sundbäck / Version 1.0 / 2020-12-28 | FRONT DS | REAR DS | RESET | GND LIGHT 4.5V | 2x I2C | 3.3V GND SCL SDA | LEFT DS | B+

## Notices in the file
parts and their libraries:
SparkFun-Connectors: Licensing: Creative Commons ShareAlike 4.0 International - https://creativecommons.org/licenses/by-sa/4.0
